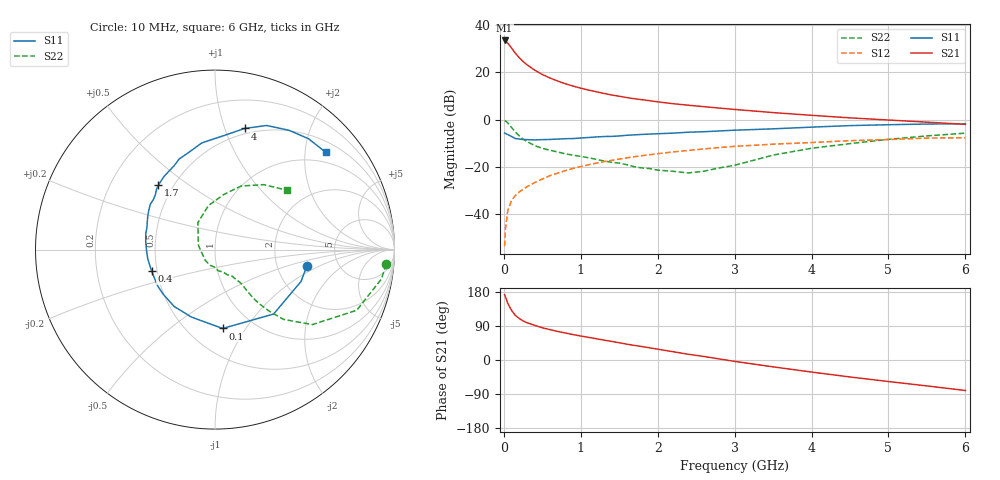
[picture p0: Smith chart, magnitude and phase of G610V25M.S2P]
! SIEMENS Small Signal Semiconductors
! BFG193
! Si NPN RF Bipolar Junction Transistor in SOT223
! VCE = 10 V  IC = 25 mA
! Common Emitter S-Parameters:  August  1996
# GHz  S  MA  R  50
!  f  S11  S21  S12  S22
! GHz  MAG  ANG  MAG  ANG  MAG  ANG  MAG  ANG
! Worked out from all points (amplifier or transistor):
!   36 points, 10 MHz to 6 GHz, reference 50 ohm
!   highest |S21| = 33.5 dB at 10 MHz (marker M1)
!   |S21| within 3 dB of that: start of sweep to 95.14 MHz
!   unconditionally stable (mu >= 1): 686.6 MHz to 2.541 GHz
!   at 250 MHz: K = 0.77, MSG = 27.1 dB, |S12| = -29.5 dB
!   at 1.4 GHz: K = 1.05, MAG = 12.5 dB, |S12| = -17.3 dB
!   at 6 GHz: K = 0.88, MSG = 2.8 dB, |S12| = -7.6 dB
!   S11 on the Smith chart (normalised r, x): 10 MHz: 2.98, -0.72; 100 MHz: 0.73, -0.79; 400 MHz: 0.47, -0.13; 1.7 GHz: 0.42, +0.39; 4 GHz: 0.45, +1.17; 6 GHz: 0.74, +2.45
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0.01  0.5207 -9.8  47.53 172.6  0.0021 83.7  0.9569 -4.9
0.02  0.5111 -20.3  46.53 167.3  0.0047 81.2  0.9419 -10.0
0.05  0.4853 -47.7  41.85 150.0  0.0117 72.4  0.8586 -23.2
0.1  0.4414 -84.5  32.87 131.1  0.0195 65.7  0.6846 -37.6
0.15  0.3982 -109.2  25.42 117.6  0.0248 60.0  0.5451 -45.5
0.2  0.3901 -125.7  20.61 109.6  0.0295 60.4  0.4555 -48.7
0.25  0.3809 -138.9  17.07 103.2  0.0336 60.8  0.3873 -50.8
0.3  0.3784 -147.7  14.59 98.4  0.038 62.1  0.3447 -51.7
0.4  0.373 -161.5  11.21 91.5  0.0465 62.4  0.2833 -52.2
0.5  0.3782 -172.3  9.039 85.1  0.0553 62.3  0.2474 -52.1
0.6  0.3815 -179.5  7.624 80.1  0.0653 62.0  0.2253 -53.0
0.7  0.3884 173.5  6.573 75.4  0.0739 61.7  0.2072 -54.6
0.9  0.3984 162.3  5.136 67.1  0.0929 59.4  0.1771 -57.0
1.1  0.4191 153.2  4.236 59.8  0.1108 56.5  0.1566 -63.9
1.4  0.4427 140.7  3.332 49.1  0.1372 51.2  0.1259 -74.9
1.7  0.4773 131.4  2.771 38.4  0.1645 45.4  0.1005 -88.8
2.2  0.519 116.2  2.178 21.9  0.2076 34.5  0.0807 -132.2
3.5  0.6397 85.0  1.412 -18.1  0.3028 4.4  0.1779 122.4
4  0.6953 76.2  1.237 -31.8  0.328 -5.1  0.2482 98.4
4.5  0.749 67.4  1.092 -44.8  0.3595 -15.2  0.3113 80.9
5.5  0.808 49.9  0.886 -68.4  0.4075 -38.4  0.4531 53.0
6  0.8211 41.4  0.797 -80.5  0.4152 -51.9  0.5186 39.7
